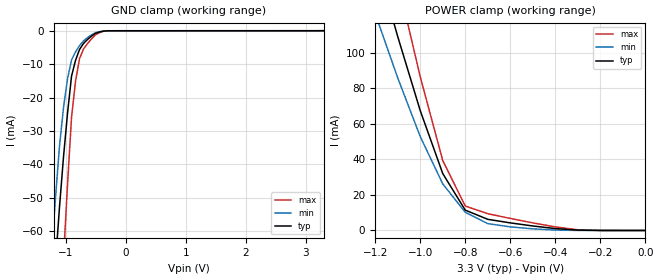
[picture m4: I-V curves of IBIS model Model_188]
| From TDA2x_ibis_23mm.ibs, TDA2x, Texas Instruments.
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| Model based on original model for IQ1833DVTCKPBFBP18LL_SSCEV
|   Sub model IQ1833_V_10P_3P3
[model]   Model_188
|[Description]  [3.3V-INPUT-X-3.3V MODE, IND, 10 PERCENT%]
|   3.3V MODE, ,IND,10 PERCENT%
|[Input Load]
|[Output Drive] 3.3V MODE
|Voltage   3.3V
|Mode   INPUT
Model_type   Input
Polarity   Non-Inverting
Vinl =  0.561
Vinh =  2.211
C_comp   469.037f   410.952f   527.122f
[Model Spec]
Vinl   0.561   0.5049   0.6171
Vinh   2.211   1.9899   2.4321
D_overshoot_ampl_h 0.66 0.66 0.66
D_overshoot_ampl_l 0.66 0.66 0.66
D_overshoot_area_h 0.33n 0.33n 0.33n
D_overshoot_area_l 0.33n 0.33n 0.33n
D_overshoot_high 3.96 3.96 3.96
D_overshoot_low -0.66 -0.66 -0.66
D_overshoot_time 1n 1n 1n
S_overshoot_high 3.3 3.3 3.3
S_overshoot_low 0 0 0
[Temperature Range]   25   125   -40
[Voltage Range]   3.3   2.97   3.63
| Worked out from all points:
|   GND clamp passes 1 mA (typ) near -0.52 V on its own axis
|   POWER clamp passes 1 mA (typ) near -0.39 V on its own axis
[POWER_clamp]
-3.3V     1.165A     1.155A     1.459A
-1.2V     153.4mA    122mA      196.7mA
-1.167V   138.6mA    109.9mA    177.9mA
-1.1V     109.1mA    85.82mA    140.3mA
-1.067V   95.17mA    74.8mA     122.3mA
-1.033V   81.28mA    63.79mA    104.4mA
-900mV    31.99mA    26.19mA    39.32mA
-800mV    11.44mA    10.22mA    13.73mA
-700mV    6.266mA    3.856mA    9.428mA
-600mV    4.272mA    2.023mA    6.777mA
-300mV    202.9uA    25.56uA    396.8uA
0V        3.057uA    1.011uA    8.442uA
[GND_clamp]
-3.3V     -675.1mA   -811.6mA   -985.9mA
-1.233V   -86.22mA   -66.38mA   -141.8mA
-1.167V   -69.2mA    -49.86mA   -116.5mA
-1.1V     -52.6mA    -34.38mA   -91.45mA
-1.033V   -37.65mA   -22.94mA   -67.83mA
-966.7mV  -24.63mA   -14.38mA   -45.95mA
-900mV    -13.56mA   -8.681mA   -25.81mA
-833.3mV  -8.843mA   -6.325mA   -15.09mA
-766.7mV  -5.582mA   -4.435mA   -8.297mA
-700mV    -3.779mA   -3.011mA   -5.442mA
-500mV    -752.8uA   -575uA     -1.188mA
3.3V      3.057uA    52.54uA    8.238uA
